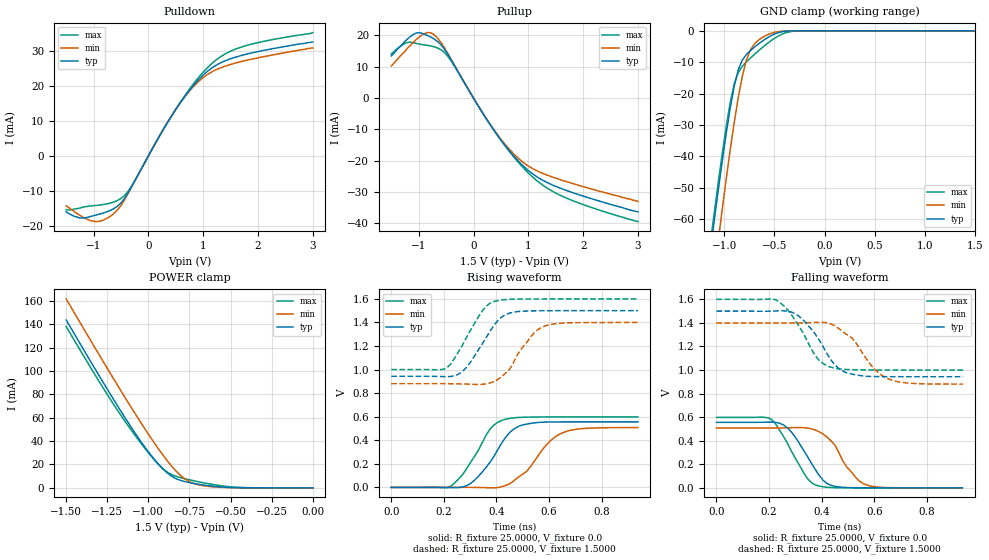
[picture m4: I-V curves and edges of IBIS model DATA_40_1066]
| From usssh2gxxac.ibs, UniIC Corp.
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|   Model DATA_40_1066
[Model]  DATA_40_1066
Model_type I/O
Polarity   Non-Inverting
Enable   Active-High
Vinl =   0.60000000V
Vinh =   0.90000000V
Vmeas =   0.750000000V
Rref =   25.00000000
Vref =   0.75000000V
C_comp   1.6160pF   1.5990pF   1.6430pF
[Temperature Range]   25.0000   95.0000   0.0
[Voltage Range]   1.5000V   1.4000V   1.6000V
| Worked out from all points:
|   slope of the pulldown table from 0 to 0.225 V, typ, clamps not added: 35.8 ohm
|   slope of the pullup table from 0 to 0.225 V, typ, clamps not added: 35.3 ohm
|   GND clamp passes 1 mA (typ) near -0.50 V on its own axis
|   POWER clamp passes 1 mA (typ) near -0.58 V on its own axis
|   rising waveform, R_fixture 25.0000, V_fixture 0.0: 20-80 % time 104ps typ, 118ps min, 96.5ps max; typ from 0 V to 0.556 V
|   rising waveform, R_fixture 25.0000, V_fixture 1.5000: 20-80 % time 96.8ps typ, 95.8ps min, 93.7ps max; typ from 0.943 V to 1.5 V
|   falling waveform, R_fixture 25.0000, V_fixture 0.0: 20-80 % time 94.1ps typ, 92.6ps min, 91.1ps max; typ from 0.556 V to 0 V
|   falling waveform, R_fixture 25.0000, V_fixture 1.5000: 20-80 % time 102ps typ, 113ps min, 95.2ps max; typ from 1.5 V to 0.943 V
[Pulldown]
|Voltage   I(typ)   I(min)   I(max)
-1.5V     -16mA      -14.3mA    -15.4mA
-1.25V    -17.76mA   -17mA      -14.93mA
-1V       -17.11mA   -18.73mA   -14.24mA
-800mV    -16.23mA   -18.22mA   -13.86mA
-600mV    -14.78mA   -16.05mA   -13mA
-350mV    -9.992mA   -10.19mA   -9.704mA
200mV     5.609mA    5.658mA    5.604mA
550mV     14.47mA    14.45mA    14.59mA
850mV     20.7mA     20.32mA    21.19mA
1.15V     25.08mA    23.98mA    26.33mA
1.75V     28.97mA    27.21mA    31.42mA
3V        32.6mA     30.9mA     35.3mA
[Pullup]
|Voltage   I(typ)   I(min)   I(max)
-1.5V     13.5mA     10.3mA     14.1mA
-1.25V    18.14mA    15mA       17.49mA
-1.05V    20.75mA    18.62mA    17.5mA
-900mV    20.45mA    20.57mA    17mA
-750mV    19.21mA    20.61mA    16.54mA
-600mV    17.13mA    17.9mA     15.49mA
-450mV    13.47mA    13.7mA     12.92mA
350mV     -9.677mA   -9.536mA   -9.657mA
900mV     -21.53mA   -20.42mA   -22.09mA
1.25V     -26.1mA    -23.92mA   -27.61mA
1.6V      -28.86mA   -26.12mA   -31.16mA
3V        -36.3mA    -33mA      -39.4mA
[GND_clamp]
|Voltage   I(typ)   I(min)   I(max)
-1.5V     -169mA     -189.1mA   -163.8mA
-1.14V    -70.71mA   -88.3mA    -68.32mA
-1.1V     -60.74mA   -77.66mA   -58.33mA
-1.06V    -51.03mA   -67.22mA   -48.61mA
-1.02V    -41.65mA   -57.06mA   -39.27mA
-940mV    -24.55mA   -37.9mA    -22.88mA
-860mV    -12.39mA   -21.26mA   -13.32mA
-780mV    -7.577mA   -9.433mA   -9.942mA
-740mV    -6.329mA   -6.125mA   -8.71mA
-620mV    -3.273mA   -2.113mA   -5.305mA
-300mV    -11.81uA   -4.878uA   -91.71uA
1.5V      4.577nA    23.6nA     33.33nA
[POWER_clamp]
|Voltage   I(typ)   I(min)   I(max)
-1.5V     143.7mA    161.7mA    138.1mA
-1.22V    77.56mA    95.29mA    73.32mA
-1.12V    55.19mA    72.34mA    52.54mA
-1.02V    34.59mA    50.23mA    33.56mA
-960mV    23.77mA    37.63mA    23.28mA
-900mV    14.66mA    25.9mA     15mA
-840mV    8.415mA    15.63mA    10.28mA
-780mV    5.408mA    7.848mA    7.861mA
-700mV    3.206mA    2.693mA    5.332mA
-600mV    1.29mA     794.5uA    2.681mA
-420mV    69.47uA    44.47uA    238.7uA
0V        4.577nA    6.249nA    39.08nA
[Ramp]
| variable   typ   min   max
dV/dt_r  0.3336/0.1041n   0.3046/0.1129n   0.3589/96.4996p
dV/dt_f  0.3342/0.1019n   0.3119/0.1089n   0.3600/95.1948p
R_load = 25.0000
[Rising Waveform]
R_fixture= 25.0000
V_fixture= 0.0
V_fixture_min= 0.0
V_fixture_max= 0.0
|time   V(typ)   V(min)   V(max)
0s        0V         0V         0V
225ps     -1.177mV   163.5uV    8.258mV
270ps     3.196mV    313.8uV    105.6mV
315ps     58.01mV    151.8uV    258.1mV
375ps     212.1mV    -3.475mV   493.1mV
435ps     426.3mV    16.64mV    579.1mV
495ps     527.9mV    105.1mV    594.7mV
590ps     554.3mV    361.8mV    597.8mV
650ps     555.7mV    462.1mV    598mV
938ps     556mV      507.7mV    598.1mV
[Rising Waveform]
R_fixture= 25.0000
V_fixture= 1.5000
V_fixture_min= 1.4000
V_fixture_max= 1.6000
|time   V(typ)   V(min)   V(max)
0s        943mV      880.2mV    1V
210ps     939.6mV    880.3mV    1.012V
255ps     959.4mV    878.8mV    1.149V
285ps     1.016V     876.9mV    1.268V
345ps     1.215V     874.4mV    1.495V
390ps     1.374V     898.2mV    1.577V
450ps     1.479V     1.003V     1.596V
495ps     1.495V     1.178V     1.599V
575ps     1.499V     1.362V     1.599V
938ps     1.5V       1.4V       1.6V
[Falling Waveform]
R_fixture= 25.0000
V_fixture= 0.0
V_fixture_min= 0.0
V_fixture_max= 0.0
|time   V(typ)   V(min)   V(max)
0s        556mV      507.7mV    598.1mV
210ps     557.8mV    507.5mV    579.3mV
255ps     534.1mV    508.9mV    436.1mV
285ps     473.9mV    510.5mV    312mV
345ps     269.6mV    508.2mV    81.51mV
390ps     107.9mV    476.9mV    15.11mV
435ps     22.07mV    400.5mV    2.952mV
495ps     2.603mV    179.2mV    333.1uV
560ps     269.1uV    34.66mV    39.72uV
935ps     0V         0V         0V
[Falling Waveform]
R_fixture= 25.0000
V_fixture= 1.5000
V_fixture_min= 1.4000
V_fixture_max= 1.6000
|time   V(typ)   V(min)   V(max)
0s        1.5V       1.4V       1.6V
225ps     1.501V     1.399V     1.597V
270ps     1.5V       1.399V     1.514V
315ps     1.455V     1.4V       1.368V
375ps     1.307V     1.404V     1.125V
435ps     1.087V     1.391V     1.024V
495ps     976.2mV    1.303V     1.004V
590ps     945.3mV    1.035V     1V
650ps     943.5mV    928.4mV    1V
938ps     943mV      880.4mV    1V
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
